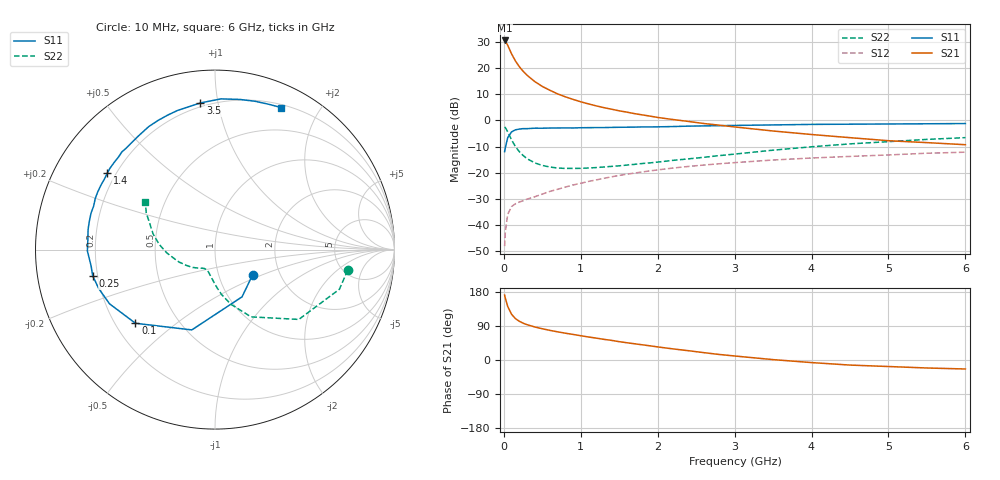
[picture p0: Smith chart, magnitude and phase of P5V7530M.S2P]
! SIEMENS Small Signal Semiconductors
! BFP183
! Si NPN RF Bipolar Junction Transistor in SOT143
! VCE = 0.75 V  IC = 30 mA
! Common Emitter S-Parameters:  March  1996
# GHz  S  MA  R  50
!  f  S11  S21  S12  S22
! GHz  MAG  ANG  MAG  ANG  MAG  ANG  MAG  ANG
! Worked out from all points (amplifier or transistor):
!   36 points, 10 MHz to 6 GHz, reference 50 ohm
!   highest |S21| = 30.7 dB at 10 MHz (marker M1)
!   |S21| within 3 dB of that: start of sweep to 68 MHz
!   unconditionally stable (mu >= 1): start of sweep to 16.67 MHz; 262.3 MHz to end of sweep
!   at 250 MHz: K = 0.97, MSG = 24.8 dB, |S12| = -30.8 dB
!   at 1.4 GHz: K = 1.71, MAG = 8.0 dB, |S12| = -21.6 dB
!   at 6 GHz: K = 1.42, MAG = -2.4 dB, |S12| = -12.2 dB
!   S11 on the Smith chart (normalised r, x): 10 MHz: 1.46, -0.43; 100 MHz: 0.28, -0.36; 250 MHz: 0.18, -0.10; 1.4 GHz: 0.17, +0.31; 3.5 GHz: 0.18, +0.89; 6 GHz: 0.23, +1.54
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0.01  0.2523 -33.6  34.12 171.3  0.0039 72.3  0.7483 -8.8
0.02  0.3033 -60.2  33.22 163.0  0.0075 69.1  0.7274 -17.7
0.05  0.4657 -106.1  27.69 141.5  0.0158 58.1  0.6078 -39.8
0.1  0.6041 -137.2  18.95 120.8  0.0224 43.4  0.4253 -61.8
0.15  0.6607 -152.8  13.87 109.3  0.0253 39.4  0.3171 -73.8
0.2  0.6832 -161.5  10.79 102.3  0.0273 39.4  0.2535 -81.6
0.25  0.697 -167.9  8.793 97.2  0.0289 39.9  0.2134 -86.8
0.3  0.6962 -172.4  7.39 93.4  0.031 42.1  0.186 -91.2
0.4  0.711 -179.4  5.594 87.2  0.0344 45.0  0.1541 -98.0
0.5  0.7104 175.7  4.485 82.5  0.0388 47.0  0.1374 -103.4
0.6  0.7159 171.0  3.782 78.1  0.0438 49.4  0.128 -107.3
0.7  0.7177 167.3  3.223 74.3  0.048 52.0  0.1226 -110.7
0.9  0.7182 160.3  2.533 67.5  0.0581 53.5  0.1206 -116.5
1.1  0.7282 153.7  2.078 60.7  0.0679 53.6  0.1228 -121.7
1.4  0.7361 144.6  1.643 51.8  0.0832 53.2  0.1319 -128.5
1.7  0.7454 136.0  1.35 42.8  0.0982 50.9  0.1442 -135.1
2.2  0.7643 123.6  1.041 29.3  0.1225 46.4  0.1719 -147.2
2.8  0.7943 109.4  0.812 14.6  0.148 39.9  0.2119 -160.8
3.5  0.8212 95.7  0.628 1.0  0.1746 32.6  0.2695 -176.1
4.5  0.848 80.6  0.468 -13.4  0.2046 21.9  0.3558 165.8
5.5  0.8635 69.6  0.376 -21.1  0.2355 12.7  0.4334 152.0
6  0.8727 65.1  0.343 -23.7  0.2466 7.6  0.4689 145.9
